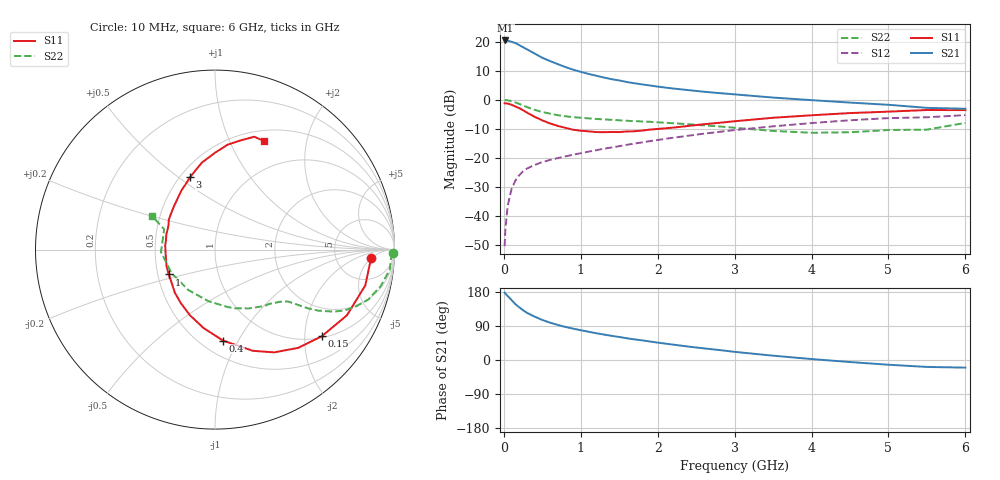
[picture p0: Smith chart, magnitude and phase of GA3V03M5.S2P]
! Infineon Technologies  Discrete & RF Semiconductors
! BF775
! Si NPN RF Bipolar Junction Transistor in SOT23
! VCE = 3 V  IC = 3.5 mA
! Common Emitter S-Parameters:  May  1996
# GHz  S  MA  R  50
!  f  S11  S21  S12  S22
! GHz  MAG  ANG  MAG  ANG  MAG  ANG  MAG  ANG
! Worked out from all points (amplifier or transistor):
!   36 points, 10 MHz to 6 GHz, reference 50 ohm
!   highest |S21| = 20.4 dB at 20 MHz (marker M1)
!   |S21| within 3 dB of that: start of sweep to 297.6 MHz
!   unconditionally stable (mu >= 1): 919 MHz to 3.688 GHz
!   at 250 MHz: K = 0.39, MSG = 21.4 dB, |S12| = -24.6 dB
!   at 1.4 GHz: K = 1.13, MAG = 9.6 dB, |S12| = -16.4 dB
!   at 6 GHz: K = 0.97, MSG = 1.1 dB, |S12| = -5.3 dB
!   S11 on the Smith chart (normalised r, x): 10 MHz: 13, -5; 150 MHz: 1.04, -2.43; 400 MHz: 0.63, -0.87; 1 GHz: 0.57, -0.17; 3 GHz: 0.56, +0.55; 6 GHz: 0.63, +1.35
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0.01  0.8725 -2.9  10.42 177.9  0.003 89.1  0.9946 -1.2
0.02  0.8659 -5.6  10.52 175.3  0.0059 87.5  0.983 -2.6
0.05  0.8607 -13.4  10.44 168.7  0.0149 83.3  0.9799 -6.6
0.1  0.8212 -26.5  9.975 158.3  0.0289 76.4  0.9452 -12.5
0.15  0.7661 -39.1  9.486 147.4  0.0405 69.0  0.8986 -18.0
0.2  0.7171 -49.8  8.749 139.2  0.05 64.5  0.8475 -21.9
0.25  0.6605 -60.1  8.038 131.3  0.0587 60.4  0.7981 -25.1
0.3  0.602 -69.5  7.417 124.5  0.0652 57.9  0.7488 -27.5
0.4  0.5093 -84.9  6.259 114.5  0.0752 53.9  0.6702 -30.5
0.5  0.4413 -98.4  5.292 105.7  0.0843 52.0  0.6155 -32.2
0.6  0.3911 -111.0  4.648 98.6  0.092 51.2  0.5752 -33.2
0.7  0.3551 -122.1  4.119 92.6  0.0986 51.2  0.5427 -34.0
0.8  0.3287 -132.8  3.663 87.3  0.1056 51.2  0.5198 -34.7
1  0.2924 -151.8  3.025 78.5  0.1201 51.6  0.4893 -36.2
1.1  0.2857 -160.9  2.793 74.6  0.1277 51.9  0.478 -37.4
1.6  0.2842 162.7  2.022 57.3  0.1675 52.5  0.4346 -43.6
2.2  0.3309 134.1  1.563 40.6  0.2217 50.5  0.3938 -54.8
3  0.4264 109.1  1.238 21.5  0.3001 44.1  0.3294 -77.0
3.5  0.4895 98.7  1.091 11.4  0.3484 38.6  0.2901 -97.1
4.5  0.5897 83.0  0.894 -5.4  0.4434 25.9  0.2753 -151.7
5.5  0.666 70.8  0.725 -18.3  0.499 10.7  0.3052 158.2
6  0.6632 65.7  0.7 -20.1  0.5443 6.5  0.4 151.7
